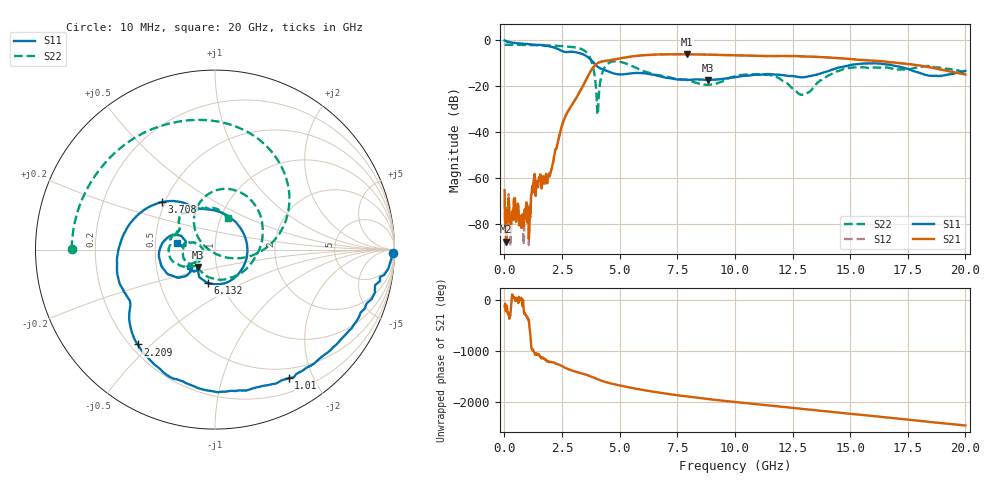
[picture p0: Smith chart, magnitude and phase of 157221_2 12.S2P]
!  2-Port S-parameters saved by WinCal
! VAR MeasName=S-Parameters (CALIBRATED_DATA) read from VNA (N5242A)
! VAR MeasDate=2015-5-26 16:47:56
! VAR NAME=157221_2 12
! VAR FILENAME=157221_2 12.S2P
! VAR DATE=2015-5-26 16:47:56
! VAR PHYS_PORTS=1,2
# Hz S DB R 50
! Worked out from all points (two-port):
!   801 points, 10 MHz to 20 GHz, reference 50 ohm
!   highest |S21| = -6.10 dB at 7.906 GHz (marker M1); lowest = -87.8 dB at 84.96 MHz (marker M2)
!   |S21| within 3 dB of the highest: 4.309 GHz to 16.32 GHz (12.01 GHz wide, 116 % of centre); 16.33814 GHz to 16.36058 GHz (22.44 MHz wide, 0.137 % of centre)
!   lowest |S11| = -17.3 dB at 8.831 GHz (marker M3), VSWR 1.32, Z = 40.5 - j8.02 ohm
!   |S11| at or under -10 dB: 3.895 GHz to end of sweep
!   |S22| runs from -32.3 to -2.0 dB; largest |S21 - S12| = 0.0099
!   S11 on the Smith chart (normalised r, x): 10 MHz: 34, -82; 1.01 GHz: 0.37, -1.67; 2.209 GHz: 0.23, -0.45; 3.708 GHz: 0.48, +0.30; 6.132 GHz: 0.86, -0.33; 20 GHz: 0.65, +0.05
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1e7  -0.07 -1.2  -65.33 -118.7  -69.72 -168.1  -1.96 179.8
8.49625e7  -0.42 -8.5  -87.77 -123.0  -85.95 84.8  -1.96 177.9
1.0095e9  -1.67 -60.2  -75.10 26.2  -74.40 29.0  -2.06 155.4
1.30935e9  -1.91 -75.9  -58.31 50.5  -58.23 51.6  -2.11 147.8
1.934038e9  -2.60 -112.9  -58.08 -130.2  -58.26 -132.6  -2.26 130.0
2.2089e9  -3.32 -129.3  -47.58 -157.1  -47.53 -157.6  -2.36 121.1
2.633688e9  -5.11 -148.4  -33.37 119.3  -33.34 119.0  -2.62 104.9
3.358325e9  -5.91 167.1  -20.81 7.8  -20.78 7.4  -3.87 62.6
3.70815e9  -8.05 137.9  -14.03 -44.2  -14.03 -44.6  -7.46 21.9
4.057975e9  -11.59 116.1  -9.88 -109.5  -9.89 -109.7  -32.19 -160.3
4.582712e9  -13.89 70.7  -8.71 175.5  -8.70 175.3  -9.60 88.5
5.382312e9  -14.60 -39.9  -7.27 96.0  -7.25 95.7  -10.58 26.8
6.131938e9  -14.44 -102.6  -6.44 33.3  -6.43 33.0  -13.72 -30.4
6.681662e9  -15.52 -122.6  -6.18 -7.0  -6.17 -7.3  -15.18 -73.5
7.90605e9  -17.14 -131.9  -6.10 -84.1  -6.09 -84.4  -17.32 -143.4
8.830588e9  -17.28 -134.7  -6.25 -135.4  -6.23 -135.8  -19.42 -148.3
1.0005e10  -16.06 -131.2  -6.55 165.8  -6.54 165.4  -15.72 -151.8
1.167916e10  -14.95 -146.2  -6.90 88.7  -6.82 88.2  -15.57 166.2
1.335332e10  -15.39 -139.5  -7.17 11.5  -7.13 11.1  -21.28 -147.0
1.505248e10  -10.72 -151.2  -8.20 -66.3  -8.18 -66.8  -11.97 -169.5
1.667666e10  -10.67 172.0  -9.48 -140.2  -9.50 -140.4  -12.00 160.7
2e10  -13.30 170.3  -14.89 66.9  -14.88 65.6  -14.35 67.8
